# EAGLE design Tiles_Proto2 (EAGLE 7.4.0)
CNAME: Tiles; CREVISION: A; DESIGNER: Simone Mora
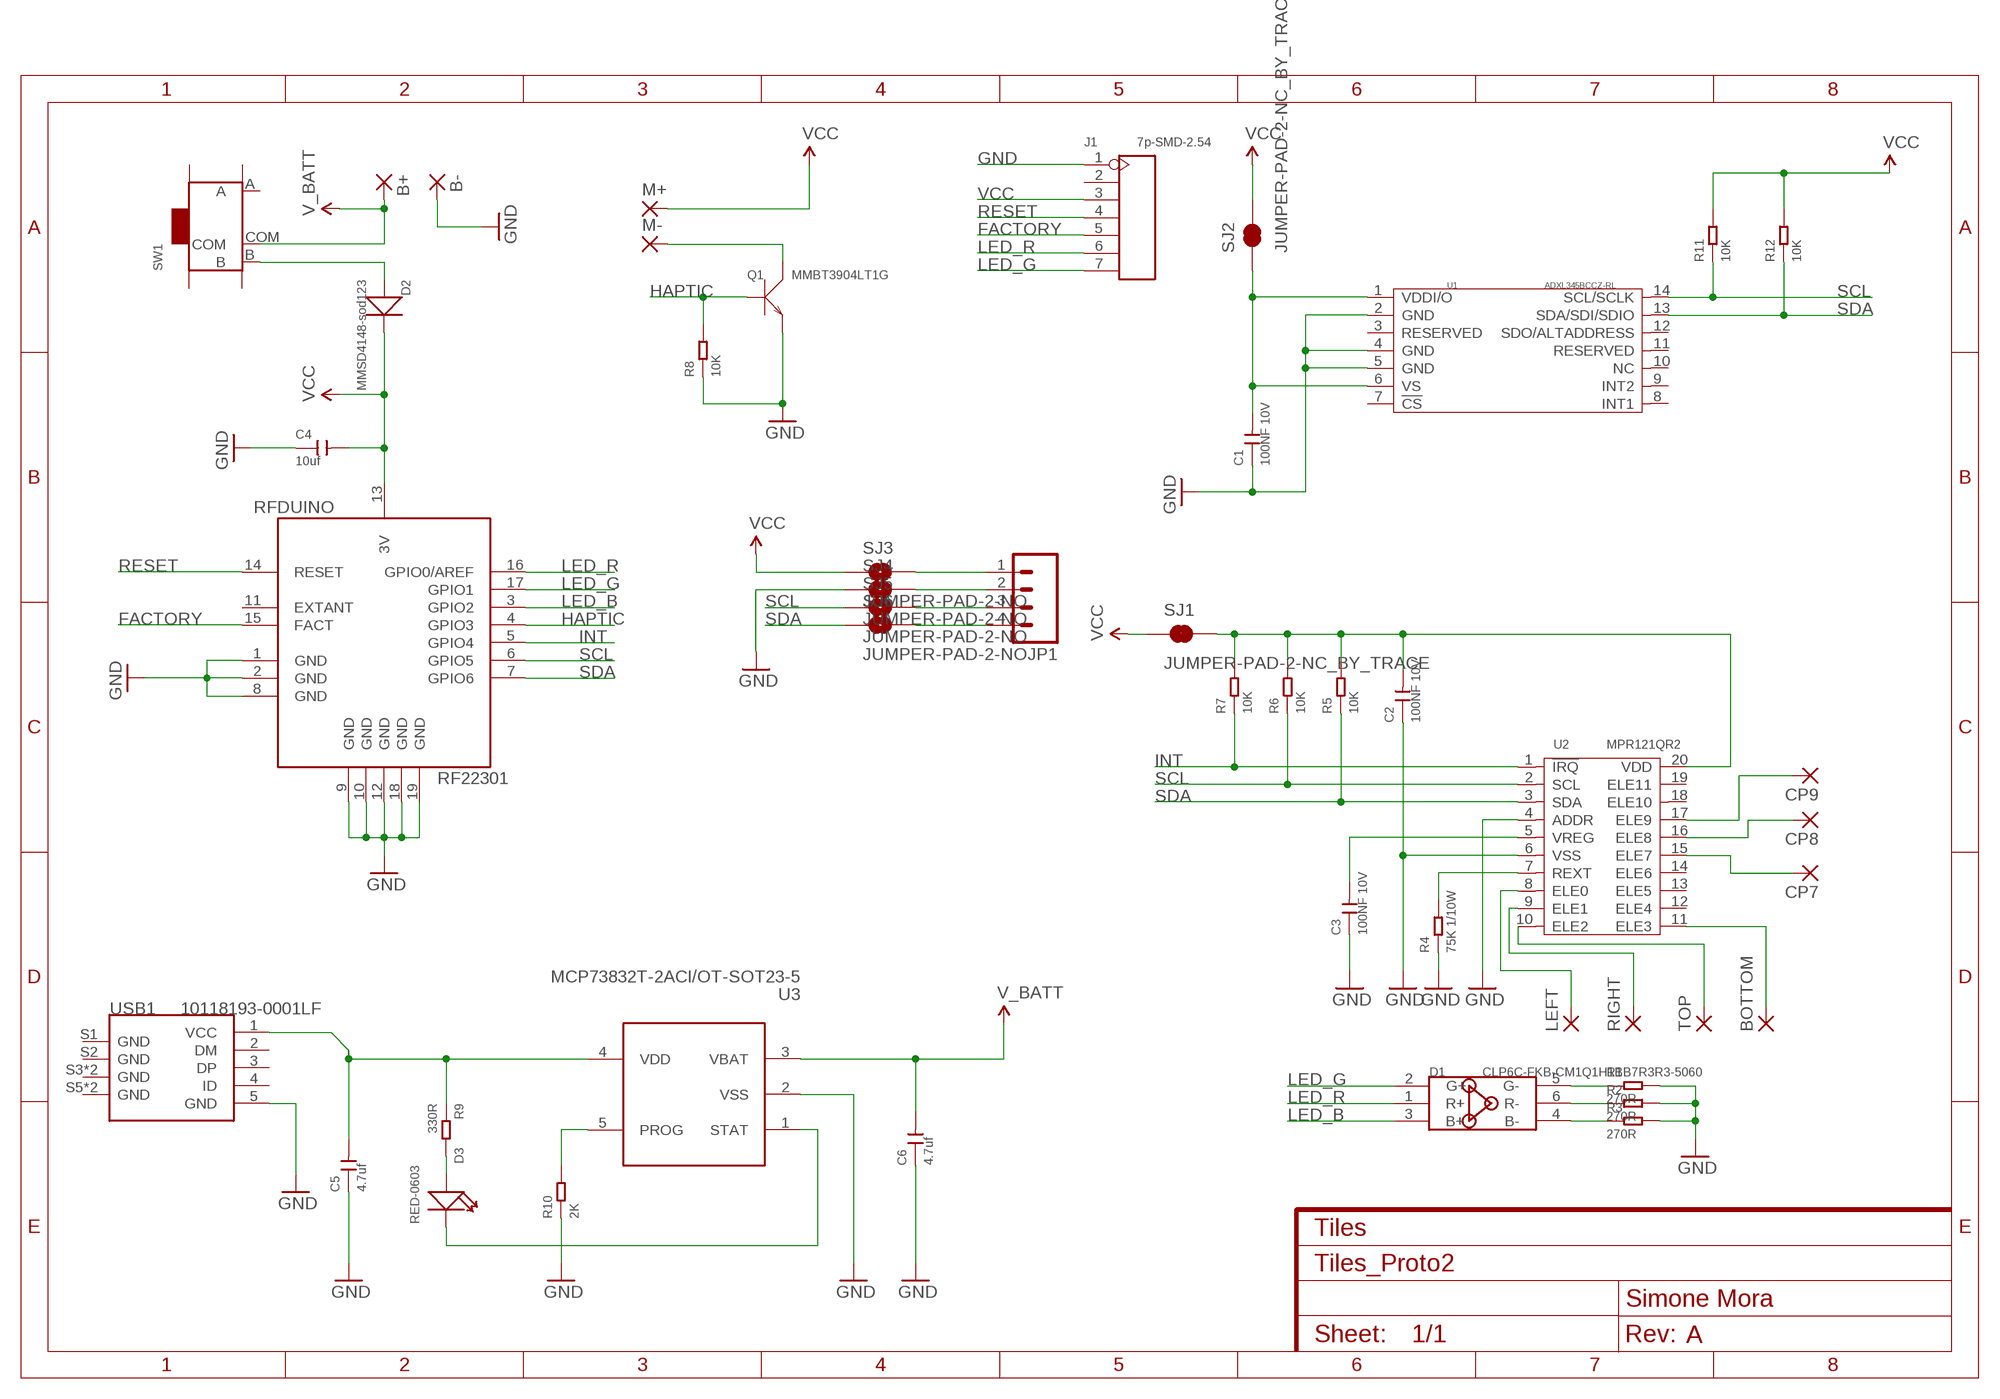
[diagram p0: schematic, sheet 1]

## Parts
B+  SMD2  [SMD1,27-2,54]
B-  SMD2  [SMD1,27-2,54]
BOTTOM  SMD5  [SMD2,54-5,08]
C1  100NF 10V  CERAMIC 100NF-10V-10%-X5R(0402)  [C0402]
C2  100NF 10V  CERAMIC 100NF-10V-10%-X5R(0402)  [C0402]
C3  100NF 10V  CERAMIC 100NF-10V-10%-X5R(0402)  [C0402]
C4  10uf  CERAMIC-10UF-6.3V-20%-X5R(0402)  [C0402]
C5  4.7uf  CERAMIC-4.7UF-6.3V-20%-X5R(0402)  [C0402]
C6  4.7uf  CERAMIC-4.7UF-6.3V-20%-X5R(0402)  [C0402]
CP7  SMD2  [SMD1,27-2,54]
CP8  SMD2  [SMD1,27-2,54]
CP9  SMD2  [SMD1,27-2,54]
D1  CLP6C-FKB-CM1Q1H1BB7R3R3-5060  SMD-LED-RGB(6P-L6.0W5.0H4.0MM)  [LED6-SMD-5060]
D2  MMSD4148-sod123  SMD-DIODE-100V-200MA(SOD-123)  [SOD-123]
D3  RED-0603  LED-SMD-RED-DIFFUSED(0603)  [LED-0603]
J1  7p-SMD-2.54  SMD-BLACK-FEMALE-HEADER(7P-2.54)  [H7-SMD-2.54]
JP1  M04PTH  [1X04]
LEFT  SMD5  [SMD2,54-5,08]
M+  SMD2  [SMD1,27-2,54]
M-  SMD2  [SMD1,27-2,54]
Q1  MMBT3904LT1G  SMD-TRANSISTORS-NPN-40V-200MA-MMBT3904LT1G(SOT-23)  [SOT-23]
R1  270R  SMD-RES-270R-5%-1/4W(1206)  [R0805]
R2  270R  SMD-RES-270R-5%-1/4W(1206)  [R0805]
R3  270R  SMD-RES-270R-5%-1/4W(1206)  [R0805]
R4  75K 1/10W  SMD-RES-75K-1%-1/10W(0603)  [R0603]
R5  10K  SMD-RES-10K-1%-1/10W(0603)  [R0603]
R6  10K  SMD-RES-10K-1%-1/10W(0603)  [R0603]
R7  10K  SMD-RES-10K-1%-1/10W(0603)  [R0603]
R8  10K  SMD-RES-10K-1%-1/10W(0603)  [R0603]
R9  330R  SMD-RES-330R-1%-1/10W(0603)  [R0603]
R10  2K  SMD-RES-2K-5%-1/10W(0603)  [R0603]
R11  10K  SMD-RES-10K-1%-1/10W(0603)  [R0603]
R12  10K  SMD-RES-10K-1%-1/10W(0603)  [R0603]
RFDUINO  RF22301  [RFD22301]
RIGHT  SMD5  [SMD2,54-5,08]
SJ1  JUMPER-PAD-2-NC_BY_TRACE  [PAD-JUMPER-2-NC_BY_TRACE_YES_SILK]
SJ2  JUMPER-PAD-2-NC_BY_TRACE  [PAD-JUMPER-2-NC_BY_TRACE_YES_SILK]
SJ3  JUMPER-PAD-2-NO  [PAD-JUMPER-2-NO_NO_SILK]
SJ4  JUMPER-PAD-2-NO  [PAD-JUMPER-2-NO_NO_SILK]
SJ5  JUMPER-PAD-2-NO  [PAD-JUMPER-2-NO_NO_SILK]
SJ6  JUMPER-PAD-2-NO  [PAD-JUMPER-2-NO_NO_SILK]
SW1  SMD-TOGGLE-SWITCH-ON-ON(3+4P-6.7X2.7MM)  [SW7-SMD-L6.7X2.7X3.2MM]
TOP  SMD5  [SMD2,54-5,08]
U1  ADXL345BCCZ-RL  MOTION/POSITION-ADXL345BCCZ-RL(14P-5.0X3.0MM)  [LGA14-0.8-5.0X3.0MM]
U2  MPR121QR2  TOUCH-MPR121QR2(QFN20)  [QFN20-0.4-3X3M]
U3  MCP73832T-2ACI/OT-SOT23-5  PMIC-MCP73832T-2ACI/OT(SOT23-5)  [SOT-23-5]
USB1  10118193-0001LF  MICRO-USB-SMD-B-(10118193-0001LF)  [MICRO-USB5+6P-SMD-0.65-B]

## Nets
FACTORY: J1.5 RFDUINO.15(FACT)
GND: B-.1(P) C1.1 C2.1 C3.1 C4.1 C5.1 C6.1 J1.1 Q1.2(E) R1.2 R2.2 R3.2 R4.1 R8.1 R10.1 RFDUINO.1(GND) RFDUINO.2(GND) RFDUINO.8(GND) RFDUINO.9(GND) RFDUINO.10(GND) RFDUINO.12(GND) RFDUINO.18(GND) RFDUINO.19(GND) SJ4.1 U1.2(GND) U1.4(GND) U1.5(GND) U2.4(ADDR) U2.6(VSS) U3.2(VSS) USB1.5(GND)
HAPTIC: Q1.1(B) R8.2 RFDUINO.4(GPIO3)
INT: R7.1 RFDUINO.5(GPIO4) U2.1(!IRQ)
LED_B: D1.3(B+) RFDUINO.3(GPIO2)
LED_G: D1.2(G+) J1.7 RFDUINO.17(GPIO1)
LED_R: D1.1(R+) J1.6 RFDUINO.16(GPIO0/AREF)
N$1: D1.5(G-) R1.1
N$2: D1.6(R-) R2.1
N$3: D1.4(B-) R3.1
N$4: C3.2 U2.5(VREG)
N$5: R4.2 U2.7(REXT)
N$6: JP1.1 SJ3.2
N$7: M-.1(P) Q1.3(C)
N$8: C5.2 R9.1 U3.4(VDD) USB1.1(VCC)
N$9: D2.+ SW1.B
N$10: D3.+ R9.2
N$11: D3.- U3.1(STAT)
N$12: R10.2 U3.5(PROG)
N$13: JP1.2 SJ4.2
N$14: JP1.3 SJ5.2
N$15: JP1.4 SJ6.2
N$16: LEFT.1(P) U2.8(ELE0)
N$17: RIGHT.1(P) U2.9(ELE1)
N$18: TOP.1(P) U2.10(ELE2)
N$19: BOTTOM.1(P) U2.11(ELE3)
N$20: CP7.1(P) U2.15(ELE7)
N$21: CP8.1(P) U2.16(ELE8)
N$22: CP9.1(P) U2.17(ELE9)
N$24: C2.2 R5.2 R6.2 R7.2 SJ1.2 U2.20(VDD)
RESET: J1.4 RFDUINO.14(RESET)
SCL: R6.1 R11.1 RFDUINO.6(GPIO5) SJ5.1 U1.14(SCL/SCLK) U2.2(SCL)
SDA: R5.1 R12.1 RFDUINO.7(GPIO6) SJ6.1 U1.13(SDA/SDI/SDIO) U2.3(SDA)
V_BATT: B+.1(P) C6.2 SW1.COM U3.3(VBAT)
VCC: C4.2 D2.- J1.3 M+.1(P) R11.2 R12.2 RFDUINO.13(3V) SJ1.1 SJ2.2 SJ3.1
VDDI/O: C1.2 SJ2.1 U1.1(VDDI/O) U1.6(VS)
Unconnected: J1.2 RFDUINO.11(EXTANT) SW1.A SW1.SS1 SW1.SS2 SW1.SS3 SW1.SS4 U1.3(RESERVED) U1.7(!CS) U1.8(INT1) U1.9(INT2) U1.10(NC) U1.11(RESERVED) U1.12(SDO/ALTADDRESS) U2.12(ELE4) U2.13(ELE5) U2.14(ELE6) U2.18(ELE10) U2.19(ELE11) USB1.2(DM) USB1.3(DP) USB1.4(ID) USB1.S1(GND) USB1.S2(GND) USB1.S3(GND) USB1.S4(GND) USB1.S5(GND) USB1.S6(GND)

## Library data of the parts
B+ B- CP7-CP9 M+ M- = wirepad:SMD2: SMD PAD
BOTTOM LEFT RIGHT TOP = wirepad:SMD5: SMD PAD
C1-C3 = Seeed-OPL-Capacitor:CERAMIC 100NF-10V-10%-X5R(0402): 302010037; MPN: CC0402KRX5R6BB104
C4 = Seeed-OPL-Capacitor:CERAMIC-10UF-6.3V-20%-X5R(0402): 302010053; MPN: CC0402MRX5R5BB106
C5 C6 = Seeed-OPL-Capacitor:CERAMIC-4.7UF-6.3V-20%-X5R(0402): 302010019; MPN: CC0402MRX5R5BB475
D1 = Seeed-OPL-Diode:SMD-LED-RGB(6P-L6.0*W5.0*H4.0MM): 304090150; MPN: CLP6C-FKB-CM1Q1H1BB7R3R3
D2 = Seeed-OPL-Diode:SMD-DIODE-100V-200MA(SOD-123): 304010007; MPN: MMSD4148
D3 = Seeed-OPL-Diode:LED-SMD-RED-DIFFUSED(0603): 304090042; MPN: 19-217-R6C-AL1M2VY-3T
J1 = Seeed-OPL-Connector:SMD-BLACK-FEMALE-HEADER(7P-2.54): 320030106; MPN: F171-1107A0BMU01
JP1 = SparkFun-Connectors:M04: Header 4 Standard 4-pin 0.1" header. Use with straight break away headers (SKU : PRT-00116), right angle break away headers (PRT-00553), swiss pins (PRT-00743), machine pins (PRT-00117), and female headers (PRT-00115). Molex polarized connector foot print use with SKU : PRT-08231 with associated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
Q1 = Seeed-OPL-Transistor:SMD-TRANSISTORS-NPN-40V-200MA-MMBT3904LT1G(SOT-23): 305010013; MPN: MMBT3904LT1G
R1-R3 = Seeed-OPL-Resistor:SMD-RES-270R-5%-1/4W(1206): 301010418; MPN: RC1206JR-07270RL
R4 = Seeed-OPL-Resistor:SMD-RES-75K-1%-1/10W(0603): 301010247; MPN: RC0603FR-0775KL
R5-R8 R11 R12 = Seeed-OPL-Resistor:SMD-RES-10K-1%-1/10W(0603): 301010299; MPN: RC0603FR-0710KL
R9 = Seeed-OPL-Resistor:SMD-RES-330R-1%-1/10W(0603): 301010300; MPN: RC0603FR-07330RL
R10 = Seeed-OPL-Resistor:SMD-RES-2K-5%-1/10W(0603): 301010113; MPN: RC0603JR-072KL
RFDUINO = GeekAmmo:RF22301: RFD22301 RFDuino Bluetooth 4.0 Low Energy BLE RF Module With Built-In ARM Cortex M0 Microconroller Hi performance, professional grade Bluetooth 4.0 Low Energy radio transceiver with built-in ARM Cortex M0 microcontroller that can be programmed using the simple-to-use Arduino IDE using RFduino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
SJ1 SJ2 = SparkFun-Passives:JUMPER-PAD-2-NC_BY_TRACE
SJ3-SJ6 = SparkFun-Passives:JUMPER-PAD-2-NO
SW1 = Seeed-OPL-Switch:SMD-TOGGLE-SWITCH-ON-ON(3+4P-6.7X2.7MM): 311030001
U1 = Seeed-OPL-sensor:MOTION/POSITION-ADXL345BCCZ-RL(14P-5.0X3.0MM): 314080008; MPN: ADXL345BCCZ-RL
U2 = Seeed-OPL-sensor:TOUCH-MPR121QR2(QFN20): 314160001; MPN: MPR121QR2
U3 = Seeed-OPL-ic:PMIC-MCP73832T-2ACI/OT(SOT23-5): 310030238; MPN: MCP73832T-2ACI/OT
USB1 = Seeed-OPL-Connector:MICRO-USB-SMD-B-(10118193-0001LF): 320010003; MPN: 10118193-0001LF

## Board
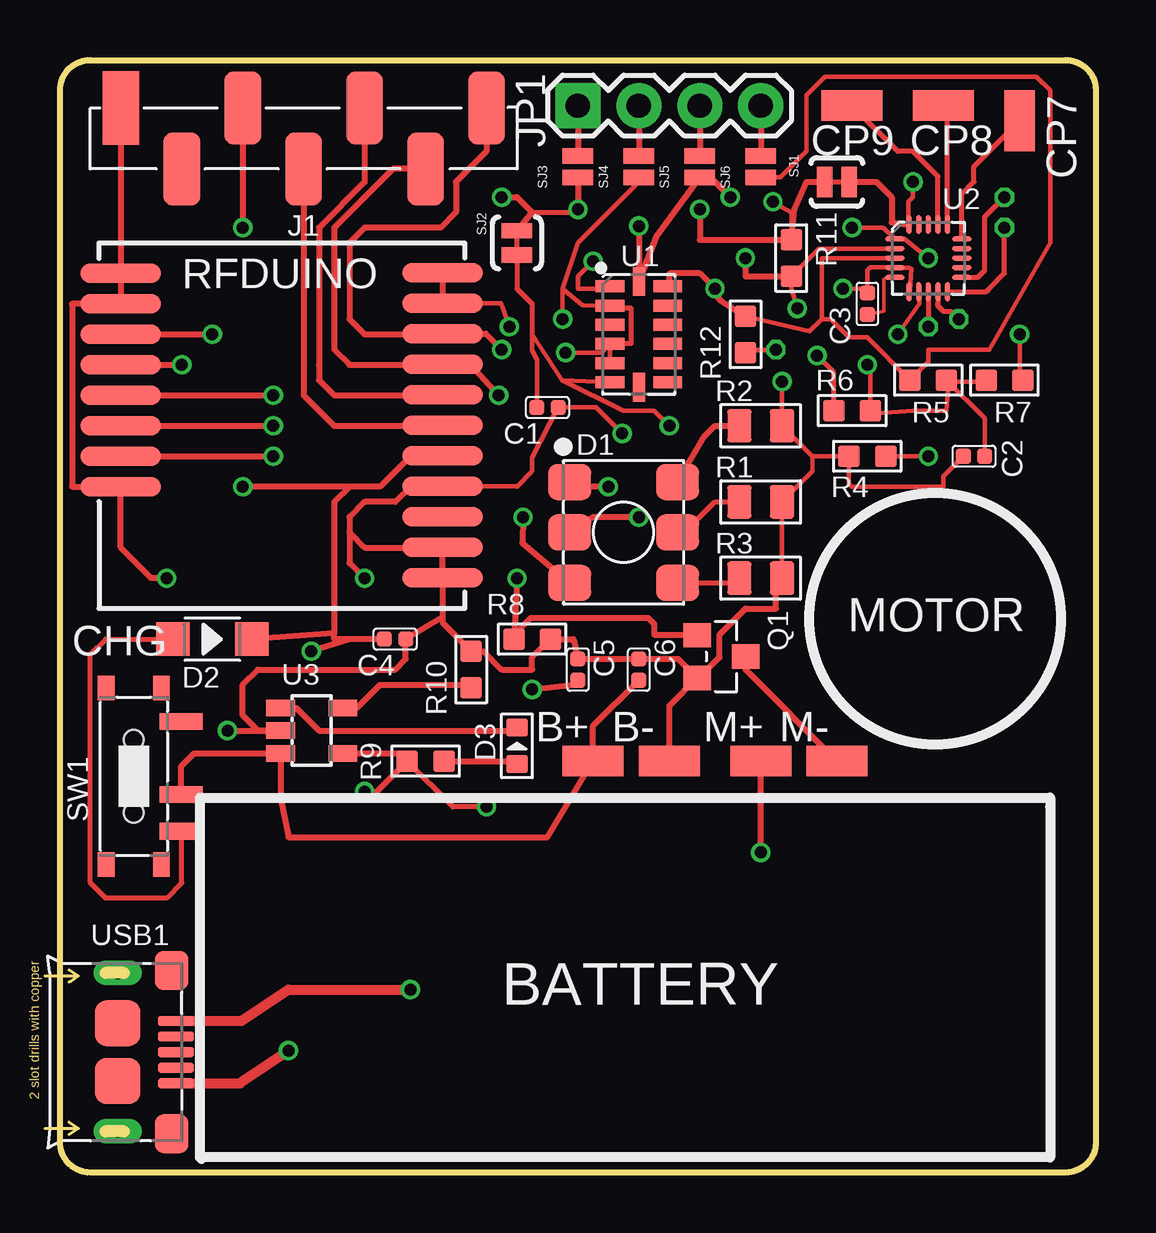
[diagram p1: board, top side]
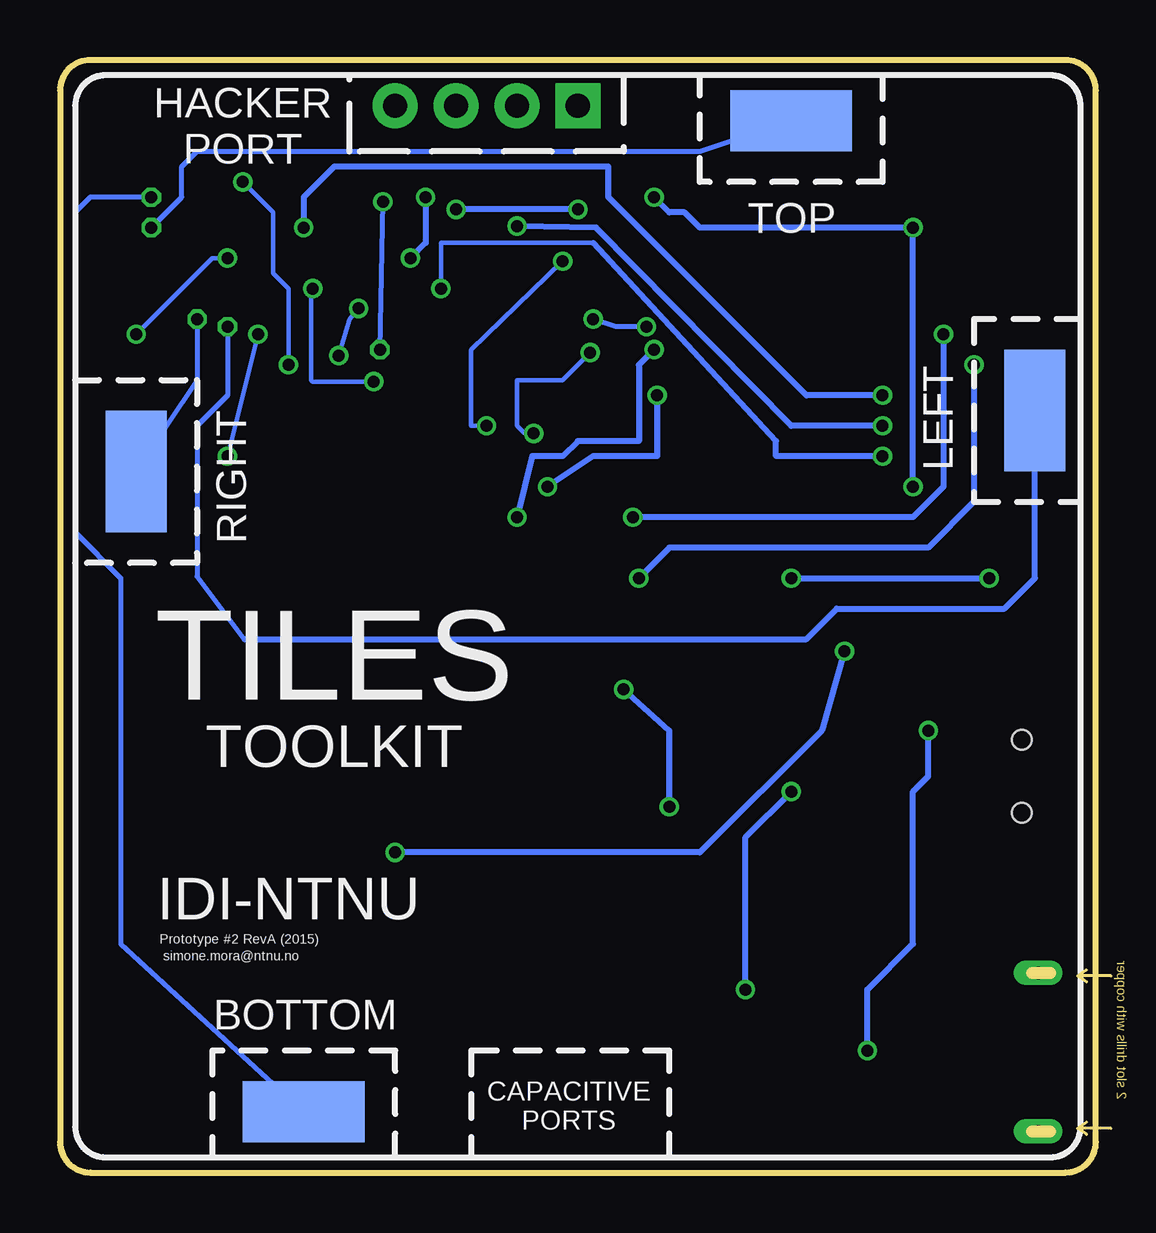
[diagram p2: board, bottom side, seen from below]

Size 43.18 x 46.36 mm. Coordinates in mm from the lower left corner, seen from the top.
Outline: 41.91,0 1.27,0 arc-90 0,1.27 0,45.08 arc-90 1.27,46.36 41.91,46.36 arc-90 43.18,45.08 43.18,1.27 arc-90 41.91,0
Copper layers (1*16): Top 0.035mm / dielectric 1.5mm / Bottom 0.035mm
Design rules "SeeedStudio_2layer_DRU_no_angle_20140221": minimum track width 6mil, minimum drill 12mil, track to track 6mil, track to pad 6mil, pad to pad 6mil, via to via 6mil, smd to smd 0mil, copper to edge 10mil, drill to drill 10mil, minimum pad ring 10mil, minimum via ring 6mil, stop-mask expansion 2mil, vias tented up to drill 100mil, thermal gap 10mil

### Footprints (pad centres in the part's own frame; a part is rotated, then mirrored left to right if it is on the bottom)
SMD1,27-2,54 = smd 1.27 x 2.54: 1 0,0
SMD2,54-5,08 = smd 2.54 x 5.08: 1 0,0
C0402 = smd 0.635 x 0.635: 1 0,0.445; 2 0,-0.445
LED6-SMD-5060 = smd 1.8 x 1.5: 1 -2.25,2.1; 2 -2.25,0; 3 -2.25,-2.1; 4 2.25,-2.1; 5 2.25,0; 6 2.25,2.1
SOD-123 = smd 1.397 x 1.397: + -1.651,0; - 1.651,0
LED-0603 = smd 0.762 x 0.889: + -0.762,0; - 0.762,0
H7-SMD-2.54 = smd 3.048 x 1.524: 1 1.27,7.62; 2 -1.27,5.08; 3 1.27,2.54; 4 -1.27,0; 5 1.27,-2.54; 6 -1.27,-5.08; 7 1.27,-7.62
1X04 = drill 1.016 pad 1.88 square: 1 0,0 | drill 1.016 pad 1.88: 2 2.54,0; 3 5.08,0; 4 7.62,0
SOT-23 = smd 1.016 x 1.143: 1 -0.889,-1.016; 2 0.889,-1.016; 3 0,1.016
R0805 = smd 1.397 x 1.016: 1 0,0.889; 2 0,-0.889
R0603 = smd 0.889 x 0.889: 1 0,0.762; 2 0,-0.762
RFD22301 = smd 3.353 x 0.813: 1 0,0; 2 0,-1.27; 3 0,-2.54; 4 0,-3.81; 5 0,-5.08; 6 0,-6.35; 7 0,-7.62; 8 0,-8.89; 9 13.411,-12.675; 10 13.411,-11.405; 11 13.411,-10.135; 12 13.411,-8.865; 13 13.411,-7.595; 14 13.411,-6.325; 15 13.411,-5.055; 16 13.411,-3.785; 17 13.411,-2.515; 18 13.411,-1.245; 19 13.411,0.025
PAD-JUMPER-2-NC_BY_TRACE_YES_SILK = smd 0.635 x 1.27: 1 -0.508,0; 2 0.508,0
PAD-JUMPER-2-NO_NO_SILK = smd 0.635 x 1.27: 1 -0.45,0; 2 0.45,0
SW7-SMD-L6.7X2.7X3.2MM = smd 1.8 x 0.7: A 1.978,2.286; B 1.978,-2.286; COM 1.978,-0.762 | smd 0.7 x 1.016: SS1 -1.15,-3.683; SS2 1.15,-3.683; SS3 1.15,3.683; SS4 -1.15,3.683 | hole 0.813: 0,-1.524; 0,1.524
LGA14-0.8-5.0X3.0MM = smd 1.2 x 0.5: 1 -1.2,2; 2 -1.2,1.2; 3 -1.2,0.4; 4 -1.2,-0.4; 5 -1.2,-1.2; 6 -1.2,-2; 8 1.2,-2; 9 1.2,-1.2; 10 1.2,-0.4; 11 1.2,0.4; 12 1.2,1.2; 13 1.2,2 | smd 0.5 x 1.2: 7 0,-2.2; 14 0,2.2
QFN20-0.4-3X3M = smd 0.8 x 0.2: 1 -1.4,0.8; 2 -1.4,0.4; 3 -1.4,0; 4 -1.4,-0.4; 5 -1.4,-0.8; 11 1.4,-0.8; 12 1.4,-0.4; 13 1.4,0; 14 1.4,0.4; 15 1.4,0.8 | smd 0.2 x 0.8: 6 -0.8,-1.4; 7 -0.4,-1.4; 8 0,-1.4; 9 0.4,-1.4; 10 0.8,-1.4; 16 0.8,1.4; 17 0.4,1.4; 18 0,1.4; 19 -0.4,1.4; 20 -0.8,1.4
SOT-23-5 = smd 0.69 x 1.2: 1 -0.95,-1.3; 2 0,-1.3; 3 0.95,-1.3; 4 0.95,1.3; 5 -0.95,1.3
MICRO-USB5+6P-SMD-0.65-B = smd 0.4 x 1.5: 1 -1.3,-0.25; 2 -0.65,-0.25; 3 0,-0.25; 4 0.65,-0.25; 5 1.3,-0.25 | smd 1.6 x 1.4: S1 -3.4,-0.427; S6 3.4,-0.427 | drill 0.508 pad 1.016 long: S2 -3.3,-2.675; S5 3.3,-2.675 | smd 1.9 x 1.9: S3 -1.2,-2.675; S4 1.2,-2.675

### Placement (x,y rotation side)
B+  22.22,17.14 270 top
B-  25.4,17.14 270 top
BOTTOM  33.02,2.54 270 bottom
C1  20.32,31.88 270 top
C2  38.1,29.84 90 top
C3  33.66,36.19 0 top
C4  13.97,22.22 270 top
C5  21.59,20.95 0 top
C6  24.13,20.95 0 top
CP7  40,43.81 0 top
CP8  36.83,44.45 90 top
CP9  33.02,44.45 90 top
D1  23.49,26.67 0 top
D2  6.35,22.22 0 top
D3  19.05,17.78 90 top
J1  10.16,43.08 90 top
JP1  21.59,44.45 0 top
LEFT  2.54,31.75 0 bottom
M+  29.21,17.14 270 top
M-  32.38,17.14 270 top
Q1  27.57,21.49 270 top
R1  29.21,27.94 90 top
R2  29.21,31.11 90 top
R3  29.21,24.77 90 top
R4  33.66,29.84 90 top
R5  36.2,33.02 90 top
R6  33.02,31.75 90 top
R7  39.37,33.02 270 top
R8  19.68,22.22 270 top
R9  15.24,17.14 90 top
R10  17.14,20.95 0 top
R11  30.48,38.1 180 top
R12  28.57,34.92 0 top
RFDUINO  2.54,37.47 0 top
RIGHT  40,29.21 0 bottom
SJ1  32.38,41.27 0 top
SJ2  19.05,38.73 90 top
SJ3  21.59,41.91 90 top
SJ4  24.13,41.91 90 top
SJ5  26.67,41.91 90 top
SJ6  29.21,41.91 90 top
SW1  3.08,16.51 0 top
TOP  12.7,43.81 90 bottom
U1  24.13,34.92 0 top
U2  36.2,38.1 0 top
U3  10.5,18.41 270 top
USB1  5.08,5.02 270 top

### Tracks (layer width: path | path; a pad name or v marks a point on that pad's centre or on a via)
FACTORY
  Top 0.254: J1.5 12.7,41.27 10.79,39.37 10.79,33.66 10.79,33.02 11.43,32.38 15.93,32.38 RFDUINO.15
GND  (via drill 0.5)
  Top 0.178: v30.1,32.96 R2.2 31.37,29.84 | v32.64,36.83 33.46,36.83 C3.1 33.66,37.59 33.78,37.72 34.78,37.72 U2.4 35.39,37.7 35.5,37.66 35.43,36.72 U2.6 | 31.37,29.84 R4.1 32.89,28.7 33.02,28.58 36.83,28.58 36.83,29.02 C2.1 | 31.37,29.84 31.37,29.21 R1.2 R3.2 | SJ4.1 24.13,41.27 22.22,39.37 21.59,38.73 20.95,36.83 | 20.95,36.83 21.78,36.13 U1.2 | U1.5 U1.4 22.57,34.16 v21.08,34.16 | RFDUINO.18 18.39,36.22 v18.73,35.24 | v20.95,35.56 20.95,36.19 20.95,36.83 | RFDUINO.12 19.02,28.6 19.05,28.58 19.68,29.21 19.68,29.78 C1.1 22.35,31.88 v23.43,30.8
  Top 0.203: 22.92,34.53 U1.4 22.95,34.54 23.81,34.54 23.81,36 23.05,36 U1.2
  Top 0.254: J1.1 RFDUINO.1 RFDUINO.2 0.51,36.19 0.51,28.58 RFDUINO.8 2.54,26.03 3.81,24.77 v4.44,24.77 | RFDUINO.19 RFDUINO.18 | RFDUINO.12 14.63,28.6 13.97,27.94 12.7,27.94 12.07,27.3 | 12.07,27.3 12.07,26.67 12.7,26.03 15.93,26.03 | 15.93,26.03 RFDUINO.10 | 15.93,26.03 15.93,24.82 RFDUINO.9 15.95,23.13 | 15.95,23.13 C4.1 14.42,21.4 13.97,20.95 8.26,20.95 7.62,20.32 7.62,19.05 8.26,18.41 U3.2 v6.99,18.41 | 12.07,27.3 12.07,25.4 v12.7,24.77 | 15.95,23.13 15.95,22.91 R10.1 17.65,21.72 18.41,20.95 19.68,20.95 19.68,21.46 R8.1 21.4,22.22 C5.1 C6.1 25.77,21.4 Q1.2 | Q1.2 26.64,20.61 27.5,21.46 27.5,22.41 28.57,23.49 29.84,23.49 29.84,24.51 R3.2 | B-.1 25.4,19.45 Q1.2
  Top 0.406: USB1.5 7.53,3.72 7.62,3.81 v9.53,5.08
  Bottom 0.178: v30.1,32.96 32.64,32.96 32.7,33.02 32.7,36.51 v32.64,36.83 | v23.43,30.8 23.81,30.8 24.13,31.11 24.13,33.02 22.22,33.02 v21.08,34.16
  Bottom 0.203: v18.73,35.24 20,35.24 v20.95,35.56
  Bottom 0.254: v12.7,24.77 v4.44,24.77 | v9.53,5.08 9.53,7.62 7.62,9.52 7.62,15.88 6.99,16.51 v6.99,18.41
HAPTIC  (via drill 0.5)
  Top 0.254: RFDUINO.4 v5.08,33.66 | v19.05,24.77 19.05,24.64 R8.2 18.92,22.41 19.62,23.11 24.51,23.11 24.77,22.86 24.77,22.41 26.53,22.41 Q1.1
  Bottom 0.254: v5.08,33.66 5.08,27.94 6.99,26.03 17.78,26.03 v19.05,24.77
INT  (via drill 0.5)
  Top 0.178: v33.02,39.37 34.32,39.37 U2.1 35.2,38.9 v36.2,38.1 | v40,34.92 40,33.15 R7.1
  Top 0.254: RFDUINO.5 v8.89,32.38
  Bottom 0.178: v36.2,38.1 36.83,38.1 v40,34.92
  Bottom 0.254: v8.89,32.38 12.07,32.38 20.32,40.64 20.32,41.91 31.75,41.91 33.02,40.64 v33.02,39.37
LED_B  (via drill 0.5)
  Top 0.254: RFDUINO.3 v6.35,34.92 | v19.3,27.3 19.27,26.22 D1.3
  Bottom 0.254: v6.35,34.92 6.35,28.58 7.62,27.3 v19.3,27.3
LED_G  (via drill 0.5)
  Top 0.254: J1.7 17.78,42.55 16.51,41.27 16.51,40 15.88,39.37 12.7,39.37 12.07,38.73 12.07,35.56 12.7,34.92 15.93,34.92 RFDUINO.17 17.75,34.95 v18.41,34.29 | v24.13,27.3 22.86,27.3 22.22,27.3 D1.2
  Bottom 0.254: v18.41,34.29 19.05,33.66 19.05,30.48 21.59,30.48 22.22,29.84 23.49,29.84 v24.13,27.3
LED_R  (via drill 0.5)
  Top 0.254: J1.6 13.88,41.81 11.43,39.37 11.43,34.29 12.07,33.66 15.93,33.66 RFDUINO.16 17.12,33.68 v18.29,32.38 | v22.86,28.58 21.44,28.58 D1.1
  Bottom 0.254: v18.29,32.38 18.29,29.84 20.32,29.84 20.95,29.84 v22.86,28.58
N$1
  Top 0.203: D1.5 26.04,26.67 27.3,27.94 R1.1
N$2
  Top 0.254: D1.6 26.86,30.67 27.3,31.11 R2.1
N$3
  Top 0.203: D1.4 28.13,24.57 R3.1
N$4
  Top 0.152: C3.2 33.59,35.75 34.35,35.88 34.35,37.21 34.42,37.27 34.77,37.27 U2.5
N$5  (via drill 0.5)
  Top 0.178: R4.2 v36.2,29.84 | v34.92,34.92 35.81,36.19 35.81,36.68 U2.7
  Bottom 0.178: v36.2,29.84 v34.92,34.92
N$6
  Top 0.254: JP1.1 SJ3.2
N$7
  Top 0.254: Q1.3 28.59,20.94 M-.1
N$8  (via drill 0.5)
  Top 0.203: v17.78,15.24 16.38,15.24 R9.1
  Top 0.254: U3.4 14.16,17.46 R9.1 13.21,15.88 v12.7,15.88 | v19.68,20.13 21.4,20.32 C5.2
  Top 0.406: USB1.1 7.59,6.32 7.62,6.35 9.53,7.62 v14.61,7.62
  Bottom 0.254: v14.61,7.62 14.61,13.97 v12.7,15.88 | v17.78,15.24 17.78,18.41 v19.68,20.13
N$9
  Top 0.203: SW1.B 5.06,12.09 5.08,12.06 4.44,11.43 1.91,11.43 1.27,12.06 1.27,21.59 1.91,22.22 D2.+
N$10
  Top 0.254: R9.2 18.92,17.14 D3.+
N$11
  Top 0.254: U3.1 9.85,19.36 10.79,18.41 18.92,18.41 D3.-
N$12
  Top 0.254: U3.5 12.38,19.36 13.34,20.32 17.02,20.32 R10.2
N$13
  Top 0.254: JP1.2 SJ4.2
N$14
  Top 0.254: JP1.3 SJ5.2
N$15
  Top 0.254: JP1.4 SJ6.2
N$16  (via drill 0.5)
  Top 0.203: U2.8 v36.2,35.24
  Bottom 0.203: v36.2,35.24 36.2,32.38 37.46,31.11 37.46,25.4 37.46,24.83 35.5,22.22
  Bottom 0.254: 35.5,22.22 12.07,22.22 10.79,23.49 3.81,23.49 2.54,24.77 LEFT.1
N$17  (via drill 0.5)
  Top 0.203: U2.9 36.59,36.21 36.58,36.19 36.58,36.13 36.83,35.88 37.15,35.88 v37.46,35.56
  Bottom 0.203: v37.46,35.56 37.46,33.02 RIGHT.1
N$18  (via drill 0.5)
  Top 0.203: U2.10 38.6,36.7 38.73,36.83 39.37,37.47 v39.37,39.37
  Bottom 0.203: v39.37,39.37 38.1,40.64 38.1,41.91 37.46,42.55 17.78,42.55 16.51,42.55 TOP.1
N$19  (via drill 0.5)
  Top 0.203: U2.11 38.25,37.3 38.55,37.59 38.55,39.81 v39.37,40.64
  Bottom 0.203: v39.37,40.64 41.91,40.64 42.55,40 42.55,26.67 40.64,24.77 40.64,9.52 BOTTOM.1
N$20
  Top 0.203: U2.15 37.59,40.77 38.1,41.27 38.1,41.91 CP7.1
N$21
  Top 0.203: U2.16 36.99,44.28 CP8.1
N$22
  Top 0.203: U2.17 36.59,41.51 36.2,41.91 35.56,42.55 34.92,42.55 CP9.1
N$24  (via drill 0.5)
  Top 0.178: 37.02,32.96 37.02,32.45 36.96,31.75 36.83,31.75 35.56,31.75 33.78,31.62 R6.2 33.78,33.53 v33.66,33.66 | 37.02,32.96 R5.2 38.55,31.43 C2.2 | v35.56,41.27 35.56,40.64 35.37,40.45 35.37,39.52 U2.20 | 37.02,32.96 38.55,32.96 R7.2
  Top 0.254: SJ1.2 33.66,41.27 34.04,41.27 34.67,40.64 34.67,39.59 U2.20
  Bottom 0.178: v33.66,33.66 33.66,36.83 34.29,37.47 34.29,40 v35.56,41.27
RESET
  Top 0.254: J1.4 10.16,35.56 10.16,32.38 11.43,31.11 15.93,31.11 RFDUINO.14
SCL  (via drill 0.5)
  Top 0.178: U2.2 31.64,38.5 R11.1 30.48,36.83 v30.73,36
  Top 0.203: R6.1 32.26,33.34 v31.56,34.04
  Top 0.254: RFDUINO.6 v8.89,31.11 | v24.13,39.43 U1.14 24.88,39.03 SJ5.1 27.12,41.46 v27.94,40.64 | v28.57,38.1 28.57,37.34 R11.1
  Bottom 0.178: v30.73,36 31.12,35.56 v31.56,34.04
  Bottom 0.254: v8.89,31.11 12.7,31.11 20.83,39.37 v24.13,39.43 | v27.94,40.64 27.94,38.73 v28.57,38.1
SDA  (via drill 0.5)
  Top 0.178: R12.1 31.24,35.05 31.75,35.56 | 31.75,35.56 31.75,38.1 U2.3 | 31.75,35.56 32.13,35.56 32.89,34.8 33.66,34.8 R5.1 36.2,33.78 36.2,34.29 37.46,34.29 38.73,34.29 41.27,38.73 41.27,45.08 40.7,45.66 31.88,45.66 31.12,44.89 31.12,42.55 30.03,41.46 SJ6.1
  Top 0.254: RFDUINO.7 v8.89,29.84 | U1.13 25.42,37.47 26.67,37.47 v27.3,36.83 27.3,36.58 27.56,36.32 R12.1
  Bottom 0.178: 20.95,38.73 27.3,38.73 v27.3,36.83
  Bottom 0.254: v8.89,29.84 13.34,29.84 13.34,30.48 20.95,38.73
V_BATT
  Top 0.254: SW1.COM 5.06,16.93 5.59,17.46 U3.3 9.2,15.57 9.53,13.97 20.32,13.97 B+.1 22.22,18.61 C6.2
VCC  (via drill 0.5)
  Top 0.203: R12.2 28.7,34.29 v29.84,34.29 | v29.72,40.45 30.48,40 R11.2 | 19.68,40 21.46,40 v21.59,40.13
  Top 0.254: J1.3 v7.62,39.37 | v18.41,40.64 19.05,40.64 19.68,40 SJ2.2 | SJ3.1 v21.59,40.13 | v26.67,40.13 26.67,38.86 R11.2 30.61,40.13 31.12,41.27 SJ1.1 | RFDUINO.13 14.63,29.87 13.34,28.58 | 13.34,28.58 v7.62,28.58 | 13.34,28.58 12.07,28.58 11.43,27.94 11.43,22.48 | 11.43,22.48 D2.- | 11.43,22.48 11.43,22.22 C4.2 12.07,22.22 v10.48,21.72 | v29.21,13.34 M+.1
  Bottom 0.203: v29.84,34.29 v29.72,40.45
  Bottom 0.254: v18.41,40.64 17.78,40 17.14,40 16.51,39.37 v7.62,39.37 v7.62,28.58 | v21.59,40.13 v26.67,40.13 | v10.48,21.72 11.43,18.41 16.51,13.34 v29.21,13.34
VDDI/O  (via drill 0.5)
  Top 0.178: 20.93,33.02 19.68,34.92 19.68,34.29 19.88,33.85 C1.2 | 20.93,33.02 U1.6 | 20.93,33.02 23.49,31.75 24.77,31.75 v25.4,31.11 | v22.22,37.97 21.59,37.34 21.59,36.83 22.83,36.83 U1.1
  Top 0.203: SJ2.1 19.05,36.83 19.68,36.19 19.68,34.92
  Bottom 0.178: v25.4,31.11 26.04,31.11 26.04,34.29 v22.22,37.97

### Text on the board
tPlace: MOTOR | CHG | BATTERY
bPlace: HACKER / PORT | TILES | TOOLKIT | IDI-NTNU | Prototype #2 RevA (2015) | simone.mora@ntnu.no | CAPACITIVE / PORTS

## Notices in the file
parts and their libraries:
SparkFun-Aesthetics: Licensing: Creative Commons ShareAlike 4.0 International - https://creativecommons.org/licenses/by-sa/4.0
